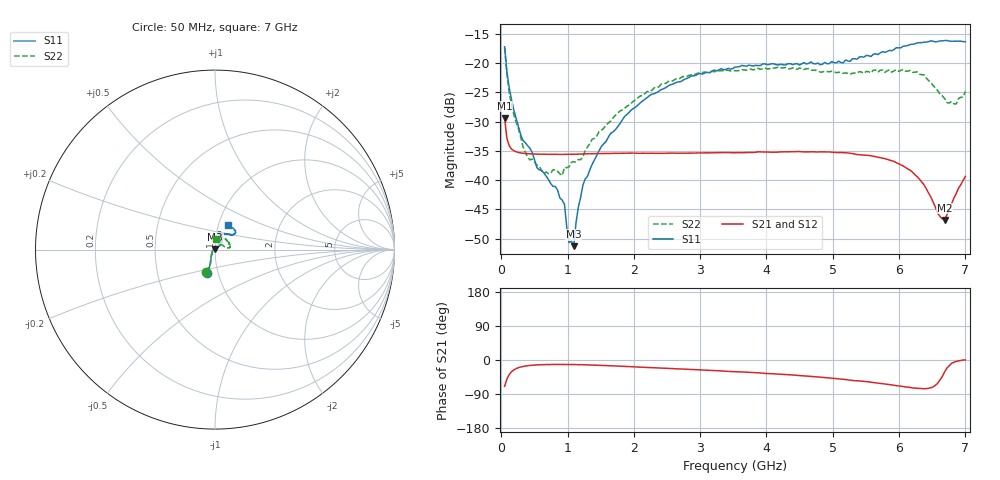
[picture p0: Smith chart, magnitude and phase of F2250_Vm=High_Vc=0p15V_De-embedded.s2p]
! Integrated Device Technology
! Corporate Headquarters
! 6024 Silver Creek Valley Road
! San Jose, CA 95138  USA
! Phone:  1-408-284-8200
! Toll Free:  1-800-223-1366
! Webpage:  http://www.idt.com/
! Timing and RF Division
! 515 Groton Road, Suite 102
! Westford, MA 01886-6024
! Device:  F2250
! Description: Voltage Variable RF Attenuator
! Frequency:  50.0 -  6000.00 MHz
! Package:  3x3 mm Thin QFN Plastic Package: 16 pin
! Ports:  2 RF, 3 DC
!  Pin  1  = GND
!  Pin  2  = NC
!  Pin  3  = RF1  = Port 1
!  Pin  4  = NC
!  Pin  5  = GND
!  Pin  6  = GND
!  Pin  7  = GND
!  Pin  8  = GND
!  Pin  9  = NC
!  Pin 10  = RF2  = Port 2
!  Pin 11  = NC
!  Pin 12  = GND
!  Pin 13  = GND
!  Pin 14  = VCNTRL
!  Pin 15  = VDD
!  Pin 16  = VMODE
! Vcntrl:  0.150 Volts
! Vmode:  +3.300 Volts
! Vdd:  +3.30  Volts
! Current:  1.243 mA
! Data:  The device was measured on a the F2250 evaluation board which has
!  individual transmission lines to the RF pins.  Data was collected
!  using a calibrated network analyzer.  The evaluation board was
!  de-embedded using a TRL calibration technique.
!  The reference plane is the edge of the package pin.
! Misc:  SN 10
!  Action Tracker AT0258
! Date Measured:  2014-11-26
! Date:  2015-10-15  MJV
! Note:
!  Integrated Device Technology supplies this data as a sample of measured
!  data at the package pin for this product.  Your particular data for this
!  product may vary.
!  Data was taken at 25 degrees C.
!  Integrated Device Technology reserves the right to change this data at anytime.
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# GHz S dB R 50
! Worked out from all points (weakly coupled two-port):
!   201 points, 50 MHz to 7 GHz, reference 50 ohm
!   highest |S21| = -29.38 dB at 50 MHz (marker M1); lowest = -46.8 dB at 6.687 GHz (marker M2)
!   lowest |S11| = -51.3 dB at 1.093 GHz (marker M3), VSWR 1.01, Z = 50 + j0.272 ohm
!   |S11| at or under -10 dB: start of sweep to end of sweep
!   |S22| runs from -39.2 to -17.4 dB; largest |S21 - S12| = 5.7e-05
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0.05  -17.18 -108.5  -29.38 -69.5  -29.38 -69.5  -17.37 -110.6
0.08475  -21.47 -107.4  -32.86 -50.1  -32.86 -50.1  -21.87 -109.0
0.15425  -26.22 -116.6  -34.68 -31.0  -34.68 -31.0  -27.10 -120.7
0.29325  -32.26 -127.5  -35.35 -18.5  -35.35 -18.4  -32.67 -133.5
0.3975  -34.12 -142.1  -35.48 -15.0  -35.48 -15.1  -36.08 -158.5
0.5365  -37.86 -154.6  -35.55 -12.9  -35.55 -12.9  -37.46 -179.9
0.64075  -38.75 -162.7  -35.58 -12.2  -35.58 -12.2  -38.87 160.5
0.91875  -43.42 155.9  -35.60 -11.8  -35.60 -11.8  -39.22 127.9
0.9535  -44.19 171.0  -35.60 -11.8  -35.60 -11.8  -37.82 124.2
1.023  -50.70 140.4  -35.59 -11.9  -35.59 -11.9  -37.71 108.0
1.0925  -51.31 90.2  -35.57 -12.0  -35.57 -12.0  -36.84 98.8
1.12725  -47.25 61.6  -35.56 -12.1  -35.56 -12.1  -36.93 91.7
1.2315  -40.85 40.9  -35.52 -12.5  -35.52 -12.5  -36.06 77.2
1.6485  -32.02 41.2  -35.44 -15.1  -35.44 -15.2  -29.92 60.0
2.37825  -24.75 46.7  -35.40 -21.0  -35.40 -21.1  -24.03 53.9
3.525  -20.65 71.7  -35.32 -30.6  -35.32 -30.6  -21.26 72.9
4.7065  -20.06 72.0  -35.15 -43.9  -35.15 -43.9  -21.21 70.4
5.85325  -17.79 40.5  -36.58 -64.8  -36.58 -64.9  -21.13 23.3
6.27025  -16.53 39.4  -39.39 -74.5  -39.40 -74.6  -21.46 8.6
6.68725  -16.11 47.9  -46.81 -31.0  -46.77 -30.8  -26.03 28.4
6.861  -16.21 54.5  -42.31 -3.7  -42.27 -3.7  -26.96 57.4
7  -16.32 62.4  -39.36 -0.1  -39.33 -0.3  -24.82 83.6
